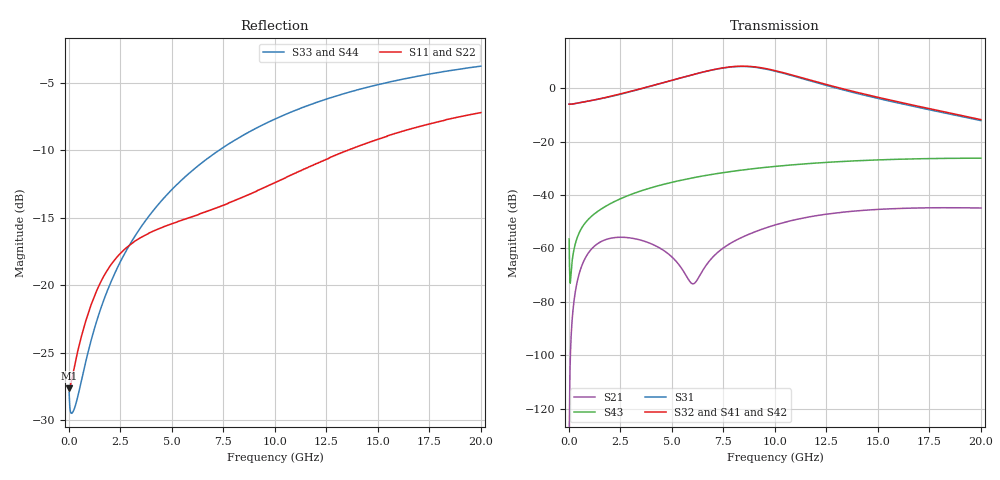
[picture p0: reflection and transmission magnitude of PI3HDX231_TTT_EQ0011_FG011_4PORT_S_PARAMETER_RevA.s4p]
! NPort=4 DATA=2000 NOISE=0 GROUPDELAY=0 COMPLEX_DATAFORMAT=POLAR
! NumOfBlock=1 NumOfParam=0
! .MODEL Smodel S TSTONEFILE=PI3HDX231_TTT_EQ0011_FG011_4PORT_S_PARAMETER_RevA.s4p TYPE=S
!  -- The above .MODEL line can be used for the S element in the netlist.
! The s parameter is extracted from the linear redriver, it is not bi-directional; only s(4,1)s(4,2) and s(3,1)s(3,2)
! should be the insertion loss
!Port definition:
!Port1 = input+
!Port2 = input-
!Port3 = output+
!Port4 = output-
# Hz S MA R  50
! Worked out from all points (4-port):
!   2000 points, 10 MHz to 20 GHz, reference 50 ohm
!   strongest paths, dB at 10 MHz, 5.01 GHz, 10.01 GHz, 15.01 GHz, 20 GHz:
!     S32: -5.9, 3.0, 6.6, -3.4, -11.8
!     S41: -5.9, 3.0, 6.6, -3.5, -11.9
!     S42: -5.9, 3.1, 6.6, -3.6, -11.7
!     S31: -5.9, 3.0, 6.4, -3.9, -12.1
!     S43: -56.5, -35.2, -29.3, -26.9, -26.2
!     S21: -134.8, -63.3, -51.2, -45.4, -44.9
!   lowest |S11| = -27.6 dB at 10 MHz (marker M1), VSWR 1.09, Z = 46 - j0.0776 ohm
!   |S11| at or under -10 dB: start of sweep to 13.55 GHz
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1e7  0.04152 -178.8  1.825e-07 -14.0  0 0.0  0 0.0
     1.825e-07 -13.9  0.04152 -178.8  0 0.0  0 0.0
     0.5041 -0.6  0.5041 179.4  0.04012 -3.2  0.0015 -70.3
     0.5041 179.4  0.5041 -0.6  0.0015 -70.3  0.04012 -3.2
5.51e9  0.1742 -139.2  0.0004002 -8.5  9.639e-10 176.5  4.334e-10 -152.7
        0.0004017 -7.6  0.1741 -139.4  4.041e-10 -151.6  1.021e-09 176.5
        1.587 -57.8  1.591 121.6  0.2466 -104.0  0.01919 58.8
        1.597 121.4  1.613 -56.7  0.01914 58.7  0.2466 -104.0
7.48e9  0.1973 -134.7  0.001006 101.2  6.751e-09 113.0  2.838e-09 -177.4
        0.001009 100.4  0.1969 -135.0  2.731e-09 -174.2  7.169e-09 111.8
        2.386 -114.5  2.404 65.1  0.3232 -109.4  0.02627 46.8
        2.41 64.9  2.434 -113.3  0.02618 46.8  0.3233 -109.4
9.02e9  0.2213 -131.3  0.00204 91.5  1.865e-08 60.9  1.211e-08 139.8
        0.002035 90.9  0.2203 -131.5  1.185e-08 142.6  1.968e-08 58.7
        2.468 -171.6  2.507 7.9  0.3789 -113.3  0.03139 36.8
        2.509 7.6  2.52 -170.4  0.03128 36.9  0.3791 -113.3
1.068e10  0.2535 -128.8  0.003244 76.2  3.825e-08 16.0  3.289e-08 82.2
          0.003232 75.8  0.2521 -129.0  3.234e-08 84.7  3.978e-08 13.0
          1.782 134.0  1.831 -46.8  0.4339 -117.3  0.03631 26.0
          1.829 -47.1  1.821 135.4  0.0362 26.2  0.434 -117.3
1.33e10  0.3112 -128.3  0.004789 49.2  9.511e-08 -39.6  8.331e-08 6.7
         0.004764 48.9  0.3092 -128.3  8.265e-08 9.2  9.689e-08 -42.7
         0.9308 75.0  0.9721 -107.1  0.5103 -123.1  0.04254 8.9
         0.967 -107.3  0.9557 76.7  0.04246 9.1  0.5103 -123.1
2e10  0.4355 -135.6  0.005737 -4.7  3.712e-07 -159.4  2.757e-07 -131.2
      0.005705 -4.8  0.4338 -135.4  2.77e-07 -129.6  3.669e-07 -162.1
      0.2472 -31.2  0.2577 142.1  0.6464 -135.0  0.0488 -32.3
      0.2554 142.4  0.2592 -29.5  0.04893 -32.0  0.6461 -135.0
